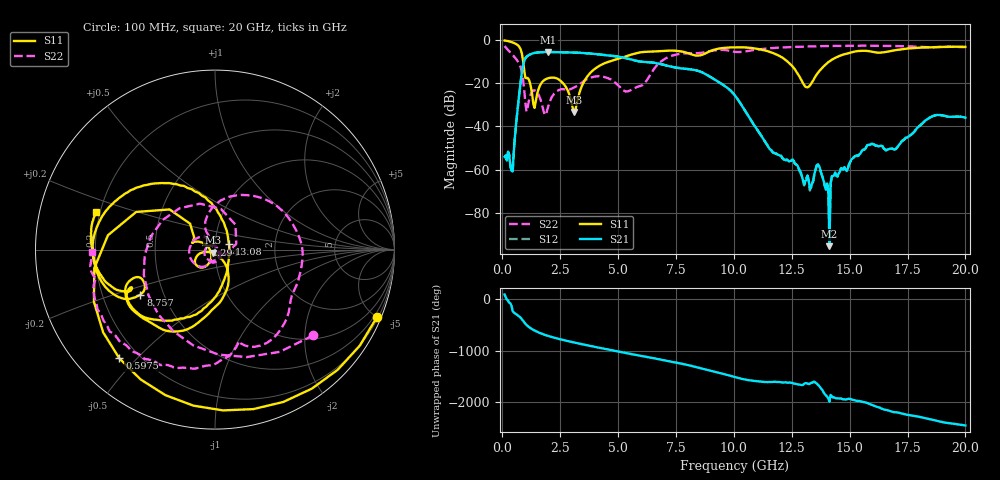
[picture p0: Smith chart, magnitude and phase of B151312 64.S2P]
!  2-Port S-parameters saved by WinCal
! VAR MeasName=S-Parameters (CALIBRATED_DATA) read from VNA (N5244A)
! VAR MeasDate=12/8/2015 5:48:49 PM
! VAR NAME=B151312 64
! VAR FILENAME=B151312 64.S2P
! VAR DATE=12/8/2015 5:48:49 PM
! VAR PHYS_PORTS=1,2
# Hz S DB R 50
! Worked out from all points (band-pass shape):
!   401 points, 100 MHz to 20 GHz, reference 50 ohm
!   highest |S21| = -5.56 dB at 1.99 GHz (marker M1); lowest = -95.4 dB at 14.13 GHz (marker M2)
!   |S21| within 3 dB of the highest: 992.3 MHz to 5.405 GHz (4.412 GHz wide, 138 % of centre)
!   lowest |S11| = -33.2 dB at 3.085 GHz (marker M3), VSWR 1.04, Z = 48.8 - j1.75 ohm
!   |S11| at or under -10 dB: 902.2 MHz to 4.611 GHz (3.708 GHz wide, 135 % of centre); 12.32 GHz to 14.11 GHz (1.791 GHz wide, 13.6 % of centre)
!   |S22| runs from -34.7 to -2.6 dB; largest |S21 - S12| = 0.0015
!   S11 on the Smith chart (normalised r, x): 100 MHz: 0.29, -4.99; 597.5 MHz: 0.13, -0.45; 1.294 GHz: 0.91, +0.04; 8.757 GHz: 0.37, -0.24; 13.08 GHz: 1.16, +0.08; 20 GHz: 0.18, +0.15
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1e8  -0.20 -22.6  -54.09 84.4  -54.07 83.0  -2.78 -41.2
3.985e8  -0.94 -87.2  -60.49 -130.9  -60.53 -132.5  -6.38 -131.2
5.975e8  -1.86 -131.3  -38.69 64.5  -38.71 64.4  -8.78 168.0
8.96e8  -9.43 138.5  -11.79 -63.0  -11.80 -63.1  -18.21 15.2
1.095e9  -17.52 163.7  -7.32 -164.4  -7.32 -164.5  -31.15 -35.9
1.294e9  -25.48 153.0  -6.25 132.4  -6.25 132.4  -23.78 -102.1
1.9905e9  -17.64 -132.0  -5.56 1.4  -5.55 1.4  -30.53 -15.6
3.085e9  -33.24 -124.4  -5.78 -123.0  -5.79 -123.0  -22.05 -110.2
3.43325e9  -21.39 -54.1  -5.97 -156.9  -5.97 -156.9  -19.69 -119.0
4.62725e9  -9.94 -89.6  -7.15 94.8  -7.13 94.8  -17.98 155.2
5.42325e9  -7.25 -104.7  -8.61 23.6  -8.59 23.5  -23.78 128.4
6.7665e9  -5.15 -135.8  -10.94 -89.5  -10.93 -89.6  -10.75 79.0
8.7565e9  -6.27 -148.9  -15.65 75.1  -15.63 75.0  -5.59 -37.6
1.005e10  -3.35 -176.7  -25.70 -75.9  -25.67 -76.3  -5.47 -75.5
1.17415e10  -6.26 130.5  -52.36 -167.2  -52.23 -168.9  -3.71 -95.5
1.308475e10  -21.58 22.8  -65.27 169.1  -66.01 165.9  -3.00 -114.7
1.338325e10  -19.41 -47.0  -66.30 175.5  -66.48 174.1  -2.99 -117.6
1.3632e10  -15.21 -72.5  -57.52 136.0  -57.69 138.4  -2.90 -121.4
1.41295e10  -9.87 -98.7  -95.39 169.3  -90.63 61.9  -2.83 -127.0
1.5821e10  -5.12 -152.6  -48.42 130.5  -48.32 130.3  -2.66 -144.8
1.67165e10  -5.24 -154.7  -50.42 -7.8  -50.36 -8.6  -2.69 -152.9
2e10  -3.17 162.5  -35.96 69.2  -36.06 68.5  -3.29 -178.8
